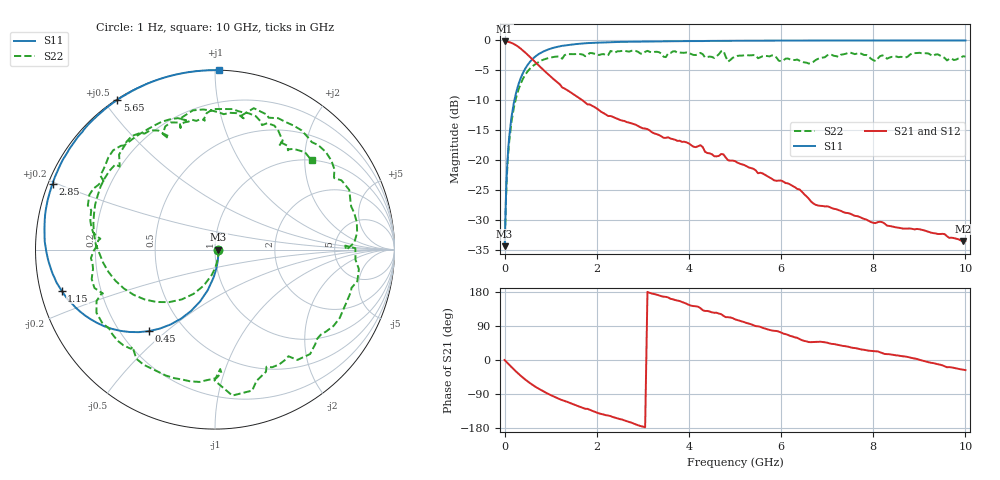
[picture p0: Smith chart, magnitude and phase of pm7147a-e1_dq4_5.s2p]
# GHz S DB R 50
! S-Parameters data
! Freq  dbS11  angS11  dbS21  angS21  dbS12  angS12  dbS22  angS22
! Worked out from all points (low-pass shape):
!   279 points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, 1 Hz to 10 GHz, reference 50 ohm
!   highest |S21| = -0.17 dB at 2.512 kHz (marker M1); lowest = -33.5 dB at 9.95 GHz (marker M2)
!   |S21| within 3 dB of the highest: start of sweep to 604.6 MHz
!   lowest |S11| = -34.3 dB at 1.259 kHz (marker M3), VSWR 1.04, Z = 52 - j0.0002 ohm
!   |S11| at or under -10 dB: start of sweep to 212.4 MHz
!   |S22| runs from -34.3 to -1.7 dB; largest |S21 - S12| = 0
!   S11 on the Smith chart (normalised r, x): 1 Hz: 1.04, -0.00; 450 MHz: 0.32, -0.44; 1.15 GHz: 0.06, -0.13; 2.85 GHz: 0.01, +0.19; 5.65 GHz: 0.00, +0.54; 10 GHz: 0.00, +1.02
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1e-09  -34.35 -0.0  -0.17 -0.0  -0.17 -0.0  -34.35 -0.0
1.2589e-06  -34.35 -0.0  -0.17 -0.0  -0.17 -0.0  -34.35 -0.0
2.5119e-06  -34.35 -0.0  -0.17 -0.0  -0.17 -0.0  -34.35 -0.0
0.06309573  -19.96 -85.2  -0.21 -8.0  -0.21 -8.0  -20.71 -87.4
0.15  -12.75 -100.2  -0.41 -18.7  -0.41 -18.7  -13.54 -107.4
0.45  -4.68 -128.9  -2.03 -51.8  -2.03 -51.8  -5.70 -150.9
0.8  -2.01 -150.7  -4.62 -80.0  -4.62 -80.0  -3.34 172.5
1.15  -1.06 -165.0  -7.02 -100.9  -7.02 -100.9  -2.69 143.4
1.7  -0.51 179.5  -10.05 -126.4  -10.05 -126.4  -2.37 105.8
2.3  -0.28 167.2  -12.62 -148.1  -12.62 -148.1  -1.76 74.7
2.85  -0.21 158.0  -14.09 -170.2  -14.09 -170.2  -1.76 37.5
3.35  -0.14 150.6  -15.79 170.4  -15.79 170.4  -1.96 6.9
4.3  -0.11 138.3  -17.81 131.4  -17.81 131.4  -2.30 -53.3
4.75  -0.07 132.9  -19.02 116.7  -19.02 116.7  -1.74 -83.2
5.05  -0.06 129.6  -20.39 105.5  -20.39 105.5  -2.59 -96.8
5.65  -0.03 123.2  -22.43 82.9  -22.43 82.9  -2.58 -137.1
6.7  -0.02 113.1  -27.21 47.4  -27.21 47.4  -3.58 173.5
7.55  -0.01 105.8  -29.10 32.1  -29.10 32.1  -2.15 132.2
8.35  -0.00 99.6  -30.97 15.2  -30.97 15.2  -2.87 105.4
9  -0.00 95.0  -31.52 0.6  -31.52 0.6  -2.06 82.9
9.95  -0.00 88.9  -33.47 -25.5  -33.47 -25.5  -2.63 47.3
10  -0.00 88.6  -33.44 -26.6  -33.44 -26.6  -2.71 42.7
